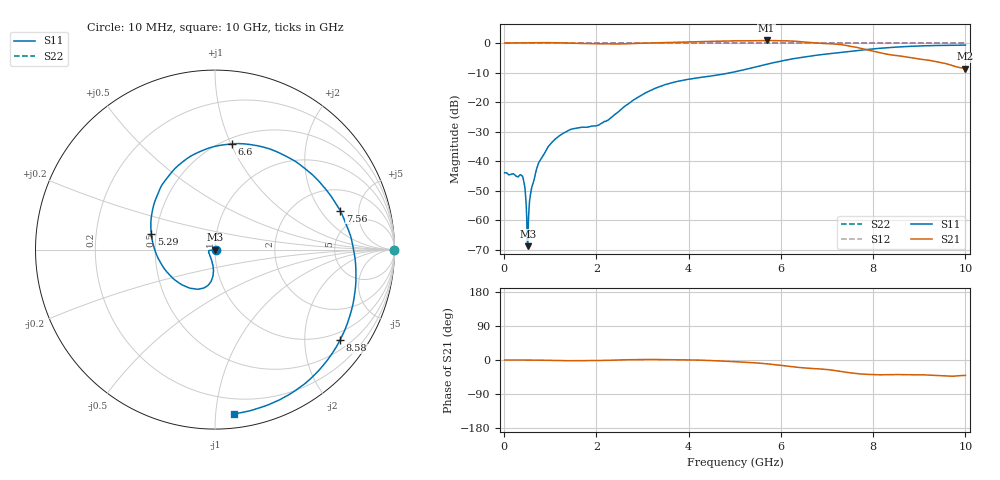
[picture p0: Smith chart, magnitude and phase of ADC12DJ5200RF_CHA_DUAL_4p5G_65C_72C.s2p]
! Texas Instruments, Inc.
! ADC12DJ5200RF - CH A S-Parameters (Dual Ch Mode, Fs = 4.5 GSPS, 65 degC case, 72 degC juntion)
! Port 1 represents the 100-ohm differenal input, Port 2 the digital output
! freq  dbS11  angS11  dbS21 angS21 dbS12 angS12 dbS22 angS22
# HZ S DB R 100
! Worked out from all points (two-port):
!   1000 points, 10 MHz to 10 GHz, reference 100 ohm
!   highest |S21| = 0.87 dB at 5.69 GHz (marker M1); lowest = -8.7 dB at 10 GHz (marker M2)
!   |S21| within 3 dB of the highest: start of sweep to 7.821 GHz
!   lowest |S11| = -68.9 dB at 510 MHz (marker M3), VSWR 1.00, Z = 100 - j0.0713 ohm
!   |S11| at or under -10 dB: start of sweep to 4.932 GHz
!   |S22| runs from 0.0 to 0.0 dB; largest |S21 - S12| = 0.76
!   S11 on the Smith chart (normalised r, x): 10 MHz: 1.01, -0.00; 5.29 GHz: 0.47, +0.10; 6.6 GHz: 0.55, +1.01; 7.56 GHz: 3.35, +3.13; 8.58 GHz: 0.75, -2.91; 10 GHz: 0.09, -1.12
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1e7  -43.98 -7.6  0.00 0.0  0.00 0.0  0.00 0.0
3.8e8  -44.92 -10.5  0.05 -0.0  0.00 0.0  0.00 0.0
4.3e8  -47.24 -0.5  0.05 -0.1  0.00 0.0  0.00 0.0
4.7e8  -52.81 6.8  0.06 -0.1  0.00 0.0  0.00 0.0
5.1e8  -68.87 -81.6  0.07 -0.1  0.00 0.0  0.00 0.0
6e8  -48.82 -136.8  0.08 -0.2  0.00 0.0  0.00 0.0
7.1e8  -42.37 -157.4  0.09 -0.3  0.00 0.0  0.00 0.0
9.4e8  -35.52 -169.1  0.12 -0.8  0.00 0.0  0.00 0.0
1.26e9  -30.80 -171.7  0.05 -1.6  0.00 0.0  0.00 0.0
1.68e9  -28.56 -163.4  -0.14 -1.8  0.00 0.0  0.00 0.0
2.24e9  -26.25 -119.8  -0.28 -0.9  0.00 0.0  0.00 0.0
3.34e9  -14.98 -96.9  0.09 1.2  0.00 0.0  0.00 0.0
4.24e9  -11.72 -125.9  0.47 -0.3  0.00 0.0  0.00 0.0
5.01e9  -9.74 -174.4  0.73 -4.6  0.00 0.0  0.00 0.0
5.29e9  -8.74 165.9  0.75 -6.2  0.00 0.0  0.00 0.0
5.69e9  -7.24 139.3  0.87 -10.1  0.00 0.0  0.00 0.0
6.6e9  -4.49 81.1  0.24 -21.7  0.00 0.0  0.00 0.0
6.67e9  -4.33 76.5  0.13 -22.4  0.00 0.0  0.00 0.0
7.56e9  -2.73 17.4  -1.21 -34.7  0.00 0.0  0.00 0.0
8.34e9  -1.56 -25.8  -3.90 -38.7  0.00 0.0  0.00 0.0
8.58e9  -1.31 -35.9  -4.39 -38.6  0.00 0.0  0.00 0.0
1e10  -0.71 -83.2  -8.71 -40.7  0.00 0.0  0.00 0.0
